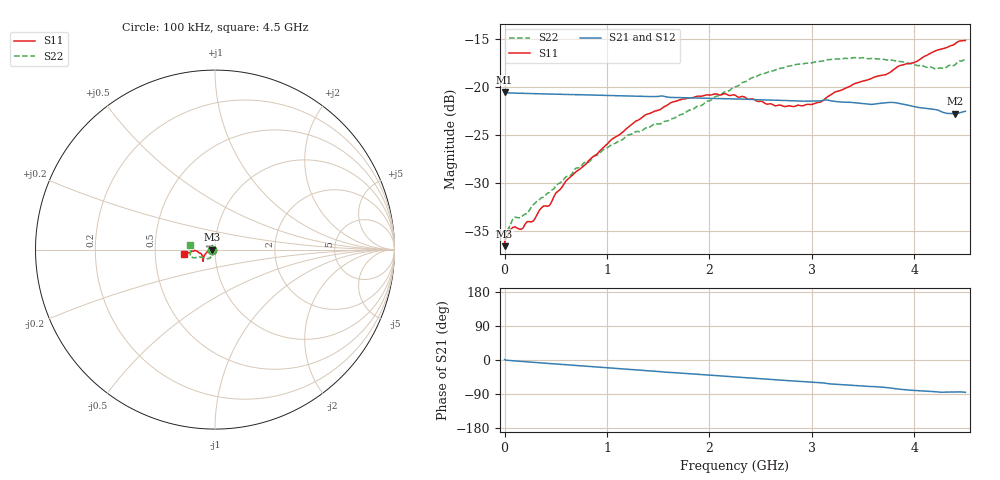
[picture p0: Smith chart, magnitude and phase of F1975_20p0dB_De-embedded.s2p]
! Integrated Device Technology
! Corporate Headquarters
! 6024 Silver Creek Valley Road
! San Jose, CA 95138  USA
! Phone:  1-408-284-8200
! Toll Free:  1-800-223-1366
! Webpage:  http://www.idt.com/
! Timing and RF Division
! 515 Groton Road, Suite 102
! Westford, MA 01886-6024
! Device:  F1975
! Description: 6-bit, 75 ohm, 0.5 dB Digital Step Attenuator
! Frequency:  5.0 MHz -  3.00 GHz
! Package:  4x4 mm QFN Plastic Package: 20 pin
! Ports:  2 RF, 11 DC
!  Pin  1  = D5 (16 dB)
!  Pin  2  = RF1  =  Port 1
!  Pin  3  = Serial Data In (DATA)
!  Pin  4  = Serial Clock (CLK)
!  Pin  5  = Serial Latch Enable (LE)
!  Pin  6  = VDD
!  Pin  7  = NC
!  Pin  8  = NC
!  Pin  9  = NC
!  Pin 10  = GND
!  Pin 11  = GND
!  Pin 12  = NC
!  Pin 13  = VMODE
!  Pin 14  = RF2  =  Port 2
!  Pin 15  = D4 (8 dB)
!  Pin 16  = D3 (4 dB)
!  Pin 17  = D2 (2 dB)
!  Pin 18  = NC
!  Pin 19  = D1 (1 dB)
!  Pin 20  = D0 (0.5 dB)
! State:  40
! Atten State:  20.0 dB
! Voltage:  +3.30 Volts
! Current:  0.593 mA
! Data:  The device was measured on a F1975 evaluation board which has
!  individual transmission lines to the RF pins.  Data was collected
!  using a calibrated network analyzer.  The evaluation board was
!  de-embedded using Automatic Fixture Removal (AFR).
!  The reference plane is the edge of the package pin.
! Misc:
!  Action Tracker AT0415
! Date Measured:  2018-02-08
! Date:  2018-03-26  MJV
! Note:
!  Integrated Device Technology supplies this data as a sample of measured
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# GHz S dB R 75
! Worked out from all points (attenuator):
!   291 points, 100 kHz to 4.5 GHz, reference 75 ohm
!   highest |S21| = -20.58 dB at 100 kHz (marker M1); lowest = -22.8 dB at 4.4 GHz (marker M2)
!   lowest |S11| = -36.6 dB at 100 kHz (marker M3), VSWR 1.03, Z = 72.8 - j0.0105 ohm
!   |S11| at or under -10 dB: start of sweep to end of sweep
!   |S22| runs from -36.2 to -17.0 dB; largest |S21 - S12| = 0.00017
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0.0001  -36.63 -179.7  -20.58 1.3  -20.57 1.2  -36.19 -178.5
0.002  -36.11 -178.4  -20.61 0.9  -20.62 0.8  -35.65 -176.9
0.01  -35.94 -178.4  -20.64 -0.4  -20.64 -0.4  -35.24 -175.2
0.08  -34.67 -175.7  -20.68 -1.9  -20.68 -1.9  -33.80 -164.1
0.16  -34.87 -176.7  -20.71 -3.6  -20.71 -3.6  -33.65 -151.0
0.22  -34.07 -178.7  -20.72 -4.9  -20.72 -4.9  -33.23 -144.3
0.28  -34.01 -179.9  -20.74 -6.1  -20.74 -6.1  -32.31 -140.7
0.36  -32.63 -179.4  -20.76 -7.7  -20.76 -7.7  -31.57 -132.9
0.44  -32.37 -178.7  -20.78 -9.3  -20.78 -9.3  -31.04 -127.2
0.6  -29.83 -174.9  -20.82 -12.5  -20.82 -12.5  -29.38 -123.0
0.76  -28.39 -168.1  -20.86 -15.7  -20.86 -15.7  -28.12 -120.7
1.28  -23.61 -152.0  -21.01 -25.9  -21.00 -25.9  -24.71 -121.5
1.52  -22.40 -144.9  -21.00 -30.4  -20.99 -30.4  -23.90 -128.5
1.88  -21.02 -138.4  -21.20 -37.5  -21.20 -37.5  -22.06 -143.5
2.26  -20.96 -137.2  -21.29 -44.7  -21.28 -44.7  -20.00 -154.8
2.64  -22.00 -147.6  -21.42 -52.0  -21.42 -52.0  -18.30 -158.3
3.02  -21.80 -164.3  -21.51 -58.8  -21.50 -58.9  -17.48 -161.1
3.42  -19.70 -175.6  -21.69 -67.6  -21.69 -67.6  -16.98 -167.1
3.76  -18.56 -175.8  -21.65 -73.7  -21.65 -73.7  -17.24 -173.7
4.2  -16.32 -172.8  -22.39 -83.6  -22.39 -83.6  -18.15 174.3
4.4  -15.55 -170.5  -22.84 -84.5  -22.84 -84.5  -17.73 171.0
4.5  -15.20 -172.2  -22.58 -85.3  -22.57 -85.3  -17.07 169.6
